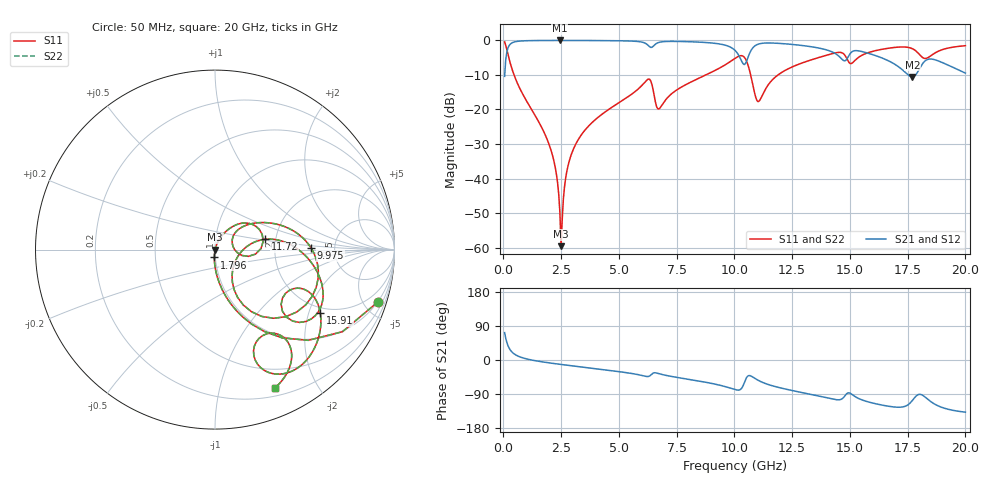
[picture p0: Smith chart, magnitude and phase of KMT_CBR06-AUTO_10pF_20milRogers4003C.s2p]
! Data measured by Modelithics Inc. support@modelithics.com 813-866-6335
! KEMET CBR06-AUTO 10pF, Pad Width= 0.851mm, Pad Length= 0.64mm, Pad Gap= 0.62mm, 20mil Rogers 4003C substrate Data, January 2022
# hz S ma R 50
! 2 Port Network Data from SP1.SP block
! freq  magS11  angS11  magS21  angS21  magS12  angS12  magS22  angS22
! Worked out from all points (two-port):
!   401 points, 50 MHz to 20 GHz, reference 50 ohm
!   highest |S21| = -0.01 dB at 2.444 GHz (marker M1); lowest = -10.6 dB at 17.71 GHz (marker M2)
!   |S21| within 3 dB of the highest: 159.8 MHz to 10.04 GHz (9.883 GHz wide, 194 % of centre); 10.71 GHz to 14.11 GHz (3.401 GHz wide, 27.4 % of centre)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
!   lowest |S11| = -59.6 dB at 2.494 GHz (marker M3), VSWR 1.00, Z = 50.1 - j0.0536 ohm
!   |S11| at or under -10 dB: 459.1 MHz to 8.761 GHz (8.302 GHz wide, 180 % of centre); 10.7 GHz to 11.89 GHz (1.183 GHz wide, 10.5 % of centre)
!   |S22| runs from -59.6 to -0.4 dB; largest |S21 - S12| = 0
!   S11 on the Smith chart (normalised r, x): 50 MHz: 0.98, -6.24; 1.796 GHz: 0.99, -0.09; 9.975 GHz: 3.30, +0.09; 11.72 GHz: 1.76, +0.22; 15.91 GHz: 1.80, -2.39; 20 GHz: 0.29, -1.49
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5e7  0.9533 -17.8  0.3017 72.2  0.3017 72.2  0.9533 -17.8
4.49e8  0.3229 -73.2  0.9459 16.7  0.9459 16.7  0.3229 -73.2
1.795625e9  0.04388 -94.8  0.9981 -6.0  0.9981 -6.0  0.04388 -94.8
2.194625e9  0.01732 -96.3  0.9988 -9.4  0.9988 -9.4  0.01732 -96.3
2.444e9  0.003197 -83.5  0.9989 -11.4  0.9989 -11.4  0.003197 -83.5
2.493875e9  0.001048 -30.7  0.9989 -11.8  0.9989 -11.8  0.001048 -30.7
2.843e9  0.01763 72.1  0.9987 -14.4  0.9987 -14.4  0.01763 72.1
3.391625e9  0.04381 69.9  0.9977 -18.5  0.9977 -18.5  0.04381 69.9
6.2345e9  0.2711 24.5  0.8668 -43.7  0.8668 -43.7  0.2711 24.5
6.73325e9  0.1018 18.3  0.9371 -36.1  0.9371 -36.1  0.1018 18.3
9.975125e9  0.5349 1.0  0.7427 -77.2  0.7427 -77.2  0.5349 1.0
1.0025e10  0.5489 -1.6  0.7176 -78.1  0.7176 -78.1  0.5489 -1.6
1.052375e10  0.5028 -49.5  0.4972 -46.4  0.4972 -46.4  0.5028 -49.5
1.10225e10  0.13 -27.4  0.8811 -53.4  0.8811 -53.4  0.13 -27.4
1.172075e10  0.2848 11.6  0.9144 -69.4  0.9144 -69.4  0.2848 11.6
1.336662e10  0.5283 -6.3  0.8065 -91.6  0.8065 -91.6  0.5283 -6.3
1.496262e10  0.4784 -39.6  0.61 -86.7  0.61 -86.7  0.4784 -39.6
1.591025e10  0.6842 -31.0  0.634 -112.4  0.634 -112.4  0.6842 -31.0
1.670825e10  0.7745 -43.5  0.4993 -122.4  0.4993 -122.4  0.7745 -43.5
1.770575e10  0.7587 -65.4  0.2951 -106.7  0.2951 -106.7  0.7587 -65.4
1.8404e10  0.5693 -54.9  0.5346 -105.2  0.5346 -105.2  0.5693 -54.9
2e10  0.8392 -66.4  0.3363 -137.6  0.3363 -137.6  0.8392 -66.4
